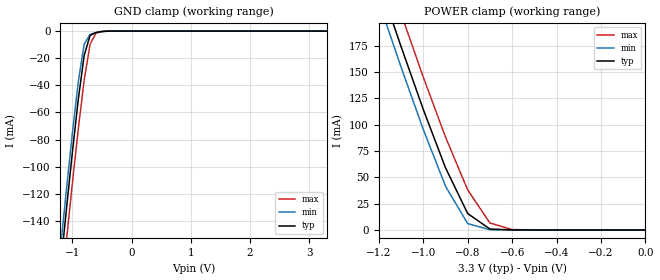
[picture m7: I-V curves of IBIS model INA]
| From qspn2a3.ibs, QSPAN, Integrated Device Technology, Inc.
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|   Model INA
[Model]   INA
Model_type   Input
Polarity   Non-Inverting
Vinl =   0.8000V
Vinh =   2.0000V
C_comp   5.00pF   5.00pF   5.00pF
[Voltage Range]   3.3000V   3.0000V   4.0000V
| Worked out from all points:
|   GND clamp passes 1 mA (typ) near -0.59 V on its own axis
|   POWER clamp passes 1 mA (typ) near -0.70 V on its own axis
[GND_clamp]
| voltage   I(typ)   I(min)   I(max)
-3.3V     -1.127A    -1.114A    -1.148A
-1.2V     -174.7mA   -160.2mA   -197.8mA
-1.1V     -131.7mA   -117.3mA   -154.8mA
-1V       -89.97mA   -75.86mA   -112.8mA
-900mV    -50.75mA   -37.66mA   -72.6mA
-800mV    -18.07mA   -9.619mA   -36.17mA
-700mV    -3.196mA   -2.415mA   -9.759mA
-600mV    -1.078mA   -1.072mA   -1.536mA
-400mV    -34.16uA   -21.02uA   -65.78uA
3.3V      8.989pA    26.27pA    105.7pA
[POWER_clamp]
| voltage   I(typ)   I(min)   I(max)
-3.3V     1.609A     1.591A     1.638A
-1.2V     235.9mA    216.5mA    267.2mA
-1.1V     174.2mA    154.7mA    205.4mA
-1V       114.5mA    95.51mA    145.2mA
-900mV    59.12mA    41.65mA    88.27mA
-800mV    15.61mA    6.061mA    38.06mA
-700mV    913.8uA    198.8uA    6.625mA
-600mV    41.62uA    9.005uA    390.5uA
0V        8.989pA    5.416pA    126.8pA
